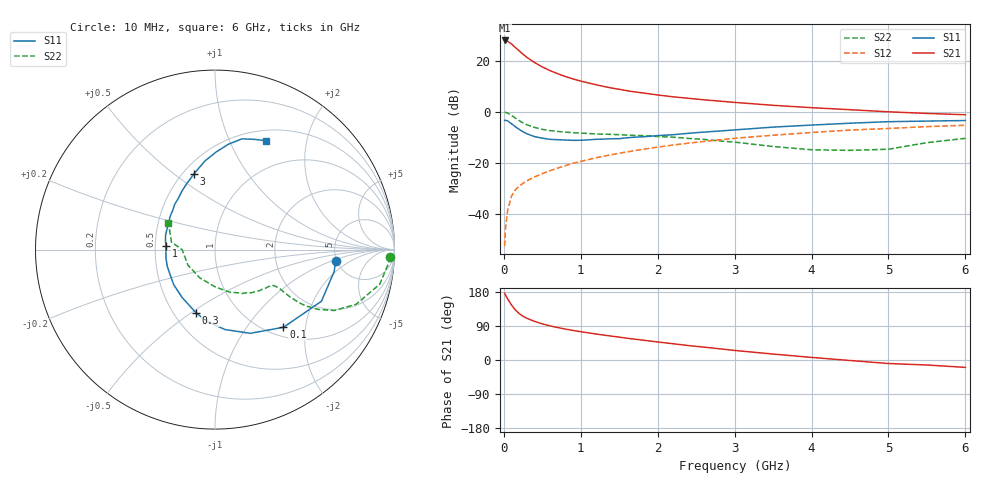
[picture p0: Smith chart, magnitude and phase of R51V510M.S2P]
! SIEMENS Small Signal Semiconductors
! BFR183
! Si NPN RF Bipolar Junction Transistor in SOT23
! VCE = 1.5 V  IC = 10 mA
! Common Emitter S-Parameters:  May  1996
# GHz  S  MA  R  50
!  f  S11  S21  S12  S22
! GHz  MAG  ANG  MAG  ANG  MAG  ANG  MAG  ANG
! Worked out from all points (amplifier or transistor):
!   36 points, 10 MHz to 6 GHz, reference 50 ohm
!   highest |S21| = 27.9 dB at 10 MHz (marker M1)
!   |S21| within 3 dB of that: start of sweep to 158.5 MHz
!   unconditionally stable (mu >= 1): 734.9 MHz to 2.535 GHz
!   at 250 MHz: K = 0.64, MSG = 25.3 dB, |S12| = -28.1 dB
!   at 1.4 GHz: K = 1.06, MAG = 11.5 dB, |S12| = -16.9 dB
!   at 6 GHz: K = 0.91, MSG = 2.1 dB, |S12| = -5.3 dB
!   S11 on the Smith chart (normalised r, x): 10 MHz: 4.87, -1.16; 100 MHz: 1.17, -1.52; 300 MHz: 0.64, -0.52; 1 GHz: 0.57, +0.03; 3 GHz: 0.57, +0.59; 6 GHz: 0.63, +1.38
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0.01  0.675 -5.5  24.89 176.2  0.0023 87.6  0.9772 -2.4
0.02  0.6752 -10.4  24.62 172.0  0.0049 85.0  0.968 -4.9
0.05  0.659 -25.9  23.91 161.0  0.0118 78.7  0.9377 -11.9
0.1  0.577 -48.6  21.22 145.0  0.0221 70.2  0.8432 -21.2
0.15  0.506 -67.2  18.07 132.0  0.0294 65.1  0.7472 -27.0
0.2  0.4488 -82.9  15.55 122.6  0.0347 62.3  0.6646 -30.1
0.25  0.4019 -96.5  13.32 115.2  0.0393 61.0  0.5991 -31.7
0.3  0.3681 -106.6  11.6 109.9  0.044 61.2  0.5531 -32.3
0.4  0.3234 -124.6  9.19 101.9  0.0525 61.7  0.4904 -32.2
0.5  0.3021 -139.6  7.518 95.2  0.0607 62.8  0.4492 -31.6
0.6  0.2866 -150.7  6.387 90.1  0.0695 63.6  0.4251 -31.2
0.7  0.2816 -160.6  5.547 85.6  0.0783 64.1  0.4095 -31.1
0.8  0.2777 -169.3  4.882 81.6  0.0873 64.3  0.3966 -31.2
1  0.2747 175.7  3.972 74.6  0.1057 64.6  0.3791 -31.9
1.1  0.2802 170.0  3.65 71.6  0.1149 64.4  0.3722 -33.2
1.6  0.3073 145.4  2.575 57.5  0.1622 61.6  0.3465 -39.1
2.2  0.3529 125.0  1.953 42.9  0.2211 56.4  0.3154 -49.6
3  0.4383 105.5  1.518 25.2  0.2999 47.4  0.2527 -70.5
3.5  0.4974 96.4  1.331 15.7  0.3448 41.0  0.207 -90.1
4.5  0.593 82.6  1.092 -1.3  0.4355 28.2  0.1739 -150.2
5.5  0.6527 70.2  0.922 -13.2  0.5081 16.1  0.2464 170.2
6  0.6695 65.0  0.869 -19.5  0.5416 8.4  0.2994 150.0
